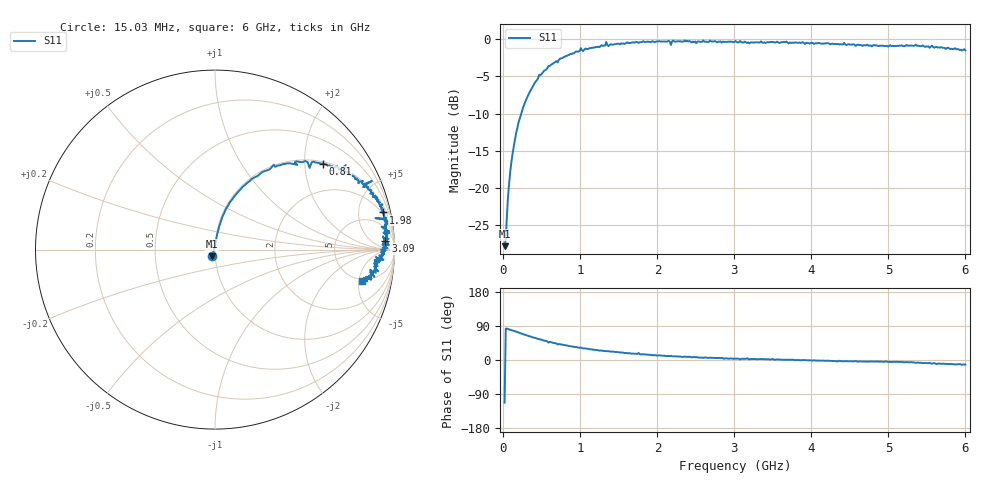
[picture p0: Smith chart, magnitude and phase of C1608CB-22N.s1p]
!	Network	Analyzer	HP8753E.07.74:	Oct	30	2002	Serial	No.	JP38451487
!	Hewlett-Packard
!	7	Sep	2009	9:39:32
!	Frequency	S11
#	HZ	S	RI	R	50
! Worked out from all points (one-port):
!   400 points, 15.03 MHz to 6 GHz, reference 50 ohm
!   lowest |S11| = -27.8 dB at 15.03 MHz (marker M1), VSWR 1.09, Z = 48.3 - j3.65 ohm
!   |S11| at or under -10 dB: start of sweep to 231.7 MHz
!   S11 on the Smith chart (normalised r, x): 15.03 MHz: 0.97, -0.07; 810 MHz: 1.05, +2.46; 1.98 GHz: 1.69, +8.84; 3.09 GHz: 19, +20; 6 GHz: 4.68, -5.55
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1.502992e7  -0.0157 -0.0377
3.002985e7  0.00555 0.0449
6.00297e7  0.0126 0.0877
1.050295e8  0.0302 0.149
1.650292e8  0.0605 0.226
2.550287e8  0.129 0.322
4.650277e8  0.327 0.473
7.650262e8  0.564 0.485
8.10026e8  0.6 0.479
1.005025e9  0.728 0.471
1.035025e9  0.715 0.421
1.320023e9  0.827 0.363
1.335023e9  0.874 0.382
1.365023e9  0.825 0.348
1.515022e9  0.865 0.311
1.755021e9  0.892 0.3
1.785021e9  0.922 0.238
1.98002e9  0.937 0.207
2.145019e9  0.955 0.177
2.175019e9  0.894 0.175
2.205019e9  0.962 0.16
2.265019e9  0.953 0.158
3.015015e9  0.967 0.0606
3.090015e9  0.949 0.0495
3.765011e9  0.941 0.00882
4.515007e9  0.916 -0.0515
5.265004e9  0.897 -0.093
6e9  0.82 -0.176
